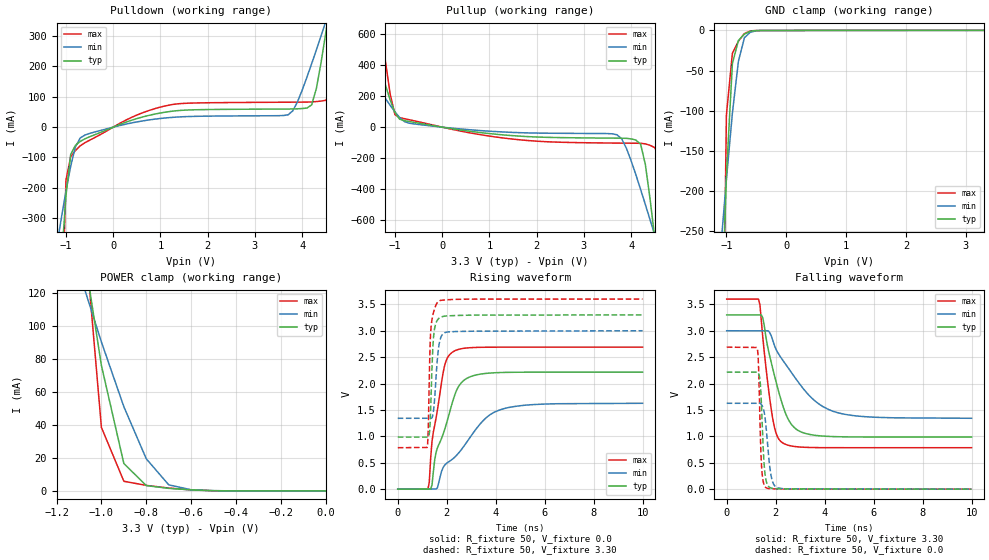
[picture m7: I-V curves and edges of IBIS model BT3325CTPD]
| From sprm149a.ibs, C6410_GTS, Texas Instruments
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[Model]   BT3325CTPD
Model_type   I/O
Vinh = 2.00
Vinl = 0.80
Enable   Active-Low
Polarity   Non-Inverting
| signals   A, GZ, Y
Vmeas = 1.5
|   typ   min   max
C_comp   1.6130p   1.5354p   1.7989p
|   typ   min   max
[Temperature Range]   25   -40   125
|   typ   min   max
[Voltage Range]   3.30V   3.00V   3.60V
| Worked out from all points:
|   slope of the pulldown table from 0 to 0.495 V, typ, clamps not added: 17.7 ohm
|   slope of the pullup table from 0 to 0.495 V, typ, clamps not added: 21.6 ohm
|   GND clamp passes 1 mA (typ) near -0.60 V on its own axis
|   POWER clamp passes 1 mA (typ) near -0.64 V on its own axis
|   rising waveform, R_fixture 50, V_fixture 0.0: 20-80 % time 839ps typ, 1.71ns min, 495ps max; typ from 0 V to 2.22 V
|   falling waveform, R_fixture 50, V_fixture 3.30: 20-80 % time 775ps typ, 1.6ns min, 432ps max; typ from 3.3 V to 0.987 V
|   rising waveform, R_fixture 50, V_fixture 3.30: 20-80 % time 116ps typ, 165ps min, 100ps max; typ from 0.987 V to 3.3 V
|   falling waveform, R_fixture 50, V_fixture 0.0: 20-80 % time 132ps typ, 209ps min, 100ps max; typ from 2.22 V to 0 V
[Pulldown]
|   Voltage   I(typ)   I(min)   I(max)
-3.3V     -6.781A    -2.576A    -22.51A
-1.1V     -449.6mA   -301.3mA   -716.1mA
-900mV    -90.06mA   -128.4mA   -97.36mA
-600mV    -38.44mA   -26.14mA   -51.28mA
1.2V      51.55mA    31.56mA    73.11mA
3.7V      59.71mA    40.51mA    82.18mA
4.2V      73.19mA    209.1mA    83.11mA
4.5V      311.7mA    348.4mA    88.34mA
4.6V      414.9mA    395.9mA    114.7mA
4.7V      520.9mA    443.6mA    265.3mA
4.8V      628.6mA    491.7mA    481.9mA
6.6V      2.64A      1.372A     5.228A
[GND_clamp]
|   Voltage   I(typ)   I(min)   I(max)
-3.3V     -6.724A    -2.539A    -22.46A
-1.1V     -408.3mA   -276.6mA   -658.2mA
-1V       -181.1mA   -185.8mA   -105.5mA
-900mV    -41.29mA   -103.1mA   -28.49mA
-800mV    -12.56mA   -38.8mA    -13.44mA
-700mV    -4.536mA   -9.108mA   -3.884mA
-600mV    -909.4uA   -2.155mA   -504.7uA
-400mV    -40.5uA    -67.44uA   -56.49uA
3.3V      100.9uA    54.24uA    177.6uA
[Pullup]
|   Voltage   I(typ)   I(min)   I(max)
-3.3V     2.594A     1.197A     5.973A
-2.2V     1.358A     659.2mA    3.014A
-1.6V     695mA      370.5mA    1.426A
-1.3V     373.6mA    230mA      661.9mA
-1V       93.8mA     98.96mA    81.06mA
-800mV    41.96mA    36.18mA    54.78mA
3.7V      -71.34mA   -49.46mA   -103.2mA
4.1V      -83.89mA   -308.7mA   -104.2mA
4.5V      -720.2mA   -699.8mA   -132.7mA
4.6V      -989mA     -800.9mA   -203.7mA
4.7V      -1.265A    -902.6mA   -740.5mA
6.6V      -6.776A    -2.885A    -19.49A
[POWER_clamp]
|   Voltage   I(typ)   I(min)   I(max)
-3.3V     2.588A     1.191A     5.971A
-1.1V     164mA      133.1mA    197.2mA
-1V       76.09mA    90.35mA    38.52mA
-900mV    16.63mA    51.09mA    5.85mA
-800mV    3.238mA    19.47mA    3.36mA
-700mV    1.562mA    3.689mA    1.736mA
-600mV    653.8uA    701.7uA    607.7uA
-500mV    154.7uA    155.6uA    89.49uA
0V        1pA        1pA        1pA
[Ramp]
|   I(typ)   I(min)   I(max)
dV/dt_r   1.330/0.841n   0.976/1.712n   1.614/0.495n
dV/dt_f   1.388/0.776n   0.995/1.604n   1.689/0.432n
[Rising Waveform]
R_fixture = 50
V_fixture = 0.0
|  pu_on
|  TIME   V(typ)   V(min)   V(max)
0s        2nV        11nV       1nV
1.233ns   2.492mV    1.667mV    1.38nV
1.288ns   2.492mV    1.85mV     130.9mV
1.399ns   77.55mV    1.85mV     902.6mV
1.566ns   696.4mV    1.85mV     1.345V
1.843ns   1.026V     398.2mV    2.177V
2.286ns   1.724V     588.7mV    2.609V
2.841ns   2.103V     904.2mV    2.675V
4.338ns   2.21V      1.525V     2.689V
10ns      2.216V     1.626V     2.689V
[Falling Waveform]
R_fixture = 50
V_fixture = 3.30
V_fixture_min = 3.00
V_fixture_max = 3.60
|  pd_on
|  TIME   V(typ)   V(min)   V(max)
0s        3.3V       3V         3.6V
1.297ns   3.3V       2.998V     3.6V
1.357ns   3.3V       2.998V     3.495V
1.477ns   3.243V     2.998V     2.866V
1.895ns   2.258V     2.797V     1.296V
2.075ns   1.93V      2.596V     992.8mV
2.314ns   1.552V     2.426V     869mV
2.912ns   1.113V     2.035V     801.1mV
4.468ns   994.2mV    1.457V     785.5mV
10ns      986.8mV    1.342V     785.2mV
[Rising Waveform]
R_fixture = 50
V_fixture = 3.30
V_fixture_min = 3.00
V_fixture_max = 3.60
|  pd_off
|  TIME   V(typ)   V(min)   V(max)
0s        986.8mV    1.342V     785.2mV
1.2ns     986.8mV    1.343V     790.5mV
1.241ns   986.8mV    1.343V     1.052V
1.302ns   1.102V     1.343V     2.376V
1.363ns   1.772V     1.343V     3.081V
1.425ns   2.585V     1.384V     3.272V
1.465ns   2.894V     1.504V     3.351V
1.69ns    3.238V     2.745V     3.564V
2.057ns   3.282V     2.978V     3.587V
10ns      3.3V       3V         3.6V
[Falling Waveform]
R_fixture = 50
V_fixture = 0.0
|  pu_off
|  TIME   V(typ)   V(min)   V(max)
0s        2.216V     1.626V     2.689V
1.251ns   2.216V     1.626V     2.655V
1.301ns   2.188V     1.626V     2.327V
1.364ns   2.052V     1.625V     1.216V
1.426ns   1.522V     1.598V     421.9mV
1.527ns   492.3mV    1.47V      83.6mV
1.615ns   152.8mV    1.145V     24.7mV
1.828ns   19.44mV    221.8mV    7.931mV
2.104ns   7.029mV    24.2mV     4.363mV
10ns      472nV      5.489uV    257.4nV
